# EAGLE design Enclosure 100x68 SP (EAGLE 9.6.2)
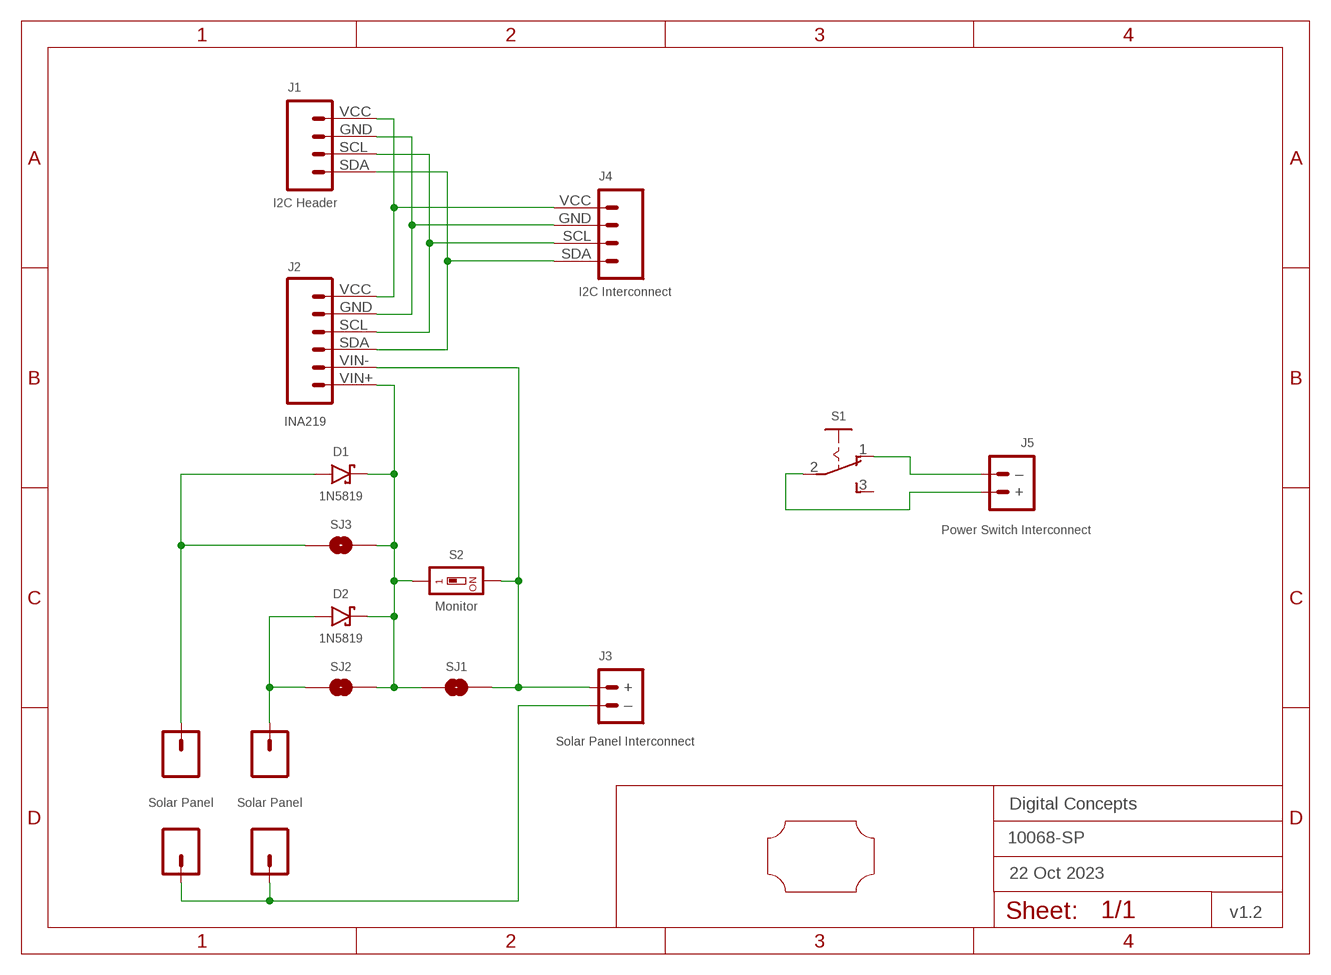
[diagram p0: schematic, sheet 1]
FRAME2 (FRAME_A5L-LOC): DATE: 22 Oct 2023; OWNER: Digital Concepts; TITLE: 10068-SP; VERSION: v1.2

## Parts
+  Solar Panel  PAD-SMD-GENERIC-SQUARE  [PAD-SMD-GENERIC]
+1  Solar Panel  PAD-SMD-GENERIC-SQUARE  [PAD-SMD-GENERIC]
-  Solar Panel  PAD-SMD-GENERIC-SQUARE  [PAD-SMD-GENERIC]
-1  Solar Panel  PAD-SMD-GENERIC-SQUARE  [PAD-SMD-GENERIC]
D1  1N5819  DIODE-SCHOTTKY-1N5819  [SOD-123]
D2  1N5819  DIODE-SCHOTTKY-1N5819  [SOD-123]
J1  I2C Header  HEADER-1X4-I2C  [CONN_04-I2C]
J2  INA219  INA219-I2C-MODULE  [CONN_06-INA219]
J3  Solar Panel Interconnect  JST-PH2.0-2-HORIZONTALJST-PTH-2  [JST-PH2.0-2-HORIZONTAL]
J4  I2C Interconnect  JST-PH2.0-4-I2C-HORIZONTAL  [JST-PH2.0-4-HORIZONTAL]
J5  Power Switch Interconnect  JST-PH2.0-2-HORIZONTALJST-PTH-2  [JST-PH2.0-2-HORIZONTAL]
S1  SWITCH-SLIDE-SPDT  [SWITCH-SPDT-PTH]
S2  Monitor  SWITCH-DIP-SWS001  [SMD-001]
SJ1  SJ  [SJ]
SJ2  SJ  [SJ]
SJ3  SJ  [SJ]
U$1  PROTO-34X22-SP  [PROTO-34X22-SP]

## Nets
GND: J1.GND J2.GND J4.GND
N$1: J1.SDA J2.SDA J4.SDA
N$2: J1.SCL J2.SCL J4.SCL
N$3: +1.P$1 D1.A SJ3.1
N$4: J2.VIN- J3.1(+) S2.2 SJ1.2
N$5: D1.C D2.C J2.VIN+ S2.1 SJ1.1 SJ2.2 SJ3.2
N$6: J5.1(+) S1.2(P)
N$7: -1.P$1 -.P$1 J3.2(–)
N$8: +.P$1 D2.A SJ2.1
N$9: J5.2(–) S1.1(O)
VCC: J1.VCC J2.VCC J4.VCC
Unconnected: S1.3(S)

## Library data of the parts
+ +1 - -1 = digitalconcepts:PAD-SMD-GENERIC-SQUARE: SMD Pad—Square
D1 D2 = digitalconcepts:DIODE-SCHOTTKY-1N5819: 1N5819 Schottky Diode SOD-123
J1 = digitalconcepts:HEADER-1X4-I2C: I2C Interface [Pin 1 Vcc] 4-Pin Header
J2 = digitalconcepts:INA219-I2C-MODULE: INA219 I2C Module
J3 J5 = digitalconcepts:JST-PH2.0-2-HORIZONTAL: PH2.0 2P Right Angle PCB Connector; PROD_ID: CONN-09863; SKU: PRT-09914
J4 = digitalconcepts:JST-PH2.0-4-I2C-HORIZONTAL: PH2.0 4P I2C Horizontal Connector
S1 = digitalconcepts:SWITCH-SLIDE-SPDT: Mini Sliding Switch SPDT
S2 = digitalconcepts:SWITCH-DIP-SWS001: SMD Dip Switch 1 pol.
SJ1-SJ3 = digitalconcepts:SJ: Solder Jumper
U$1 = digitalconcepts:PROTO-34X22-SP: 34 x 22 Prototyping board to fit an 100 x 68 enclosure—Solar panel support

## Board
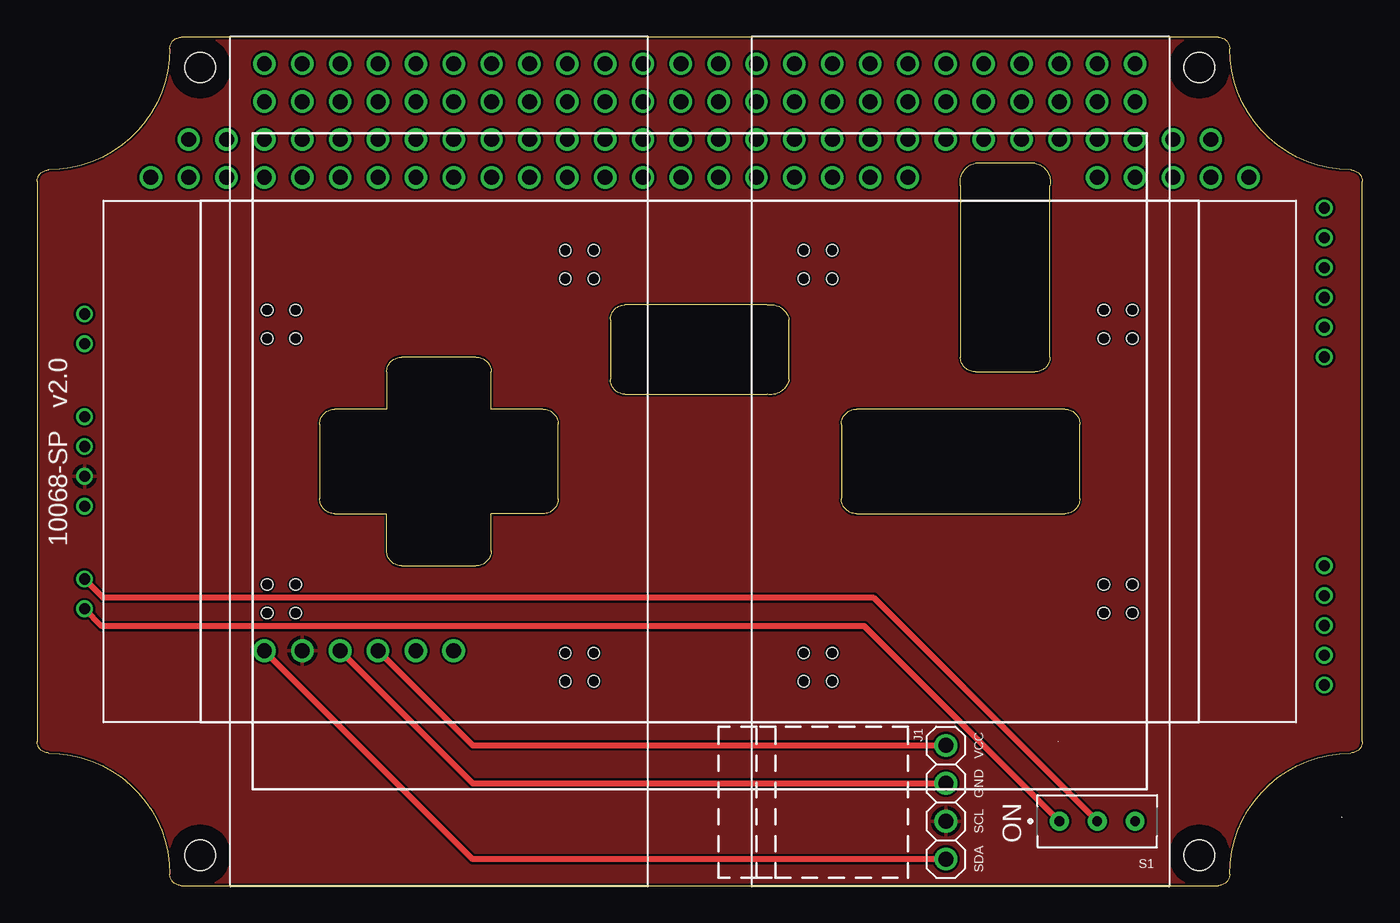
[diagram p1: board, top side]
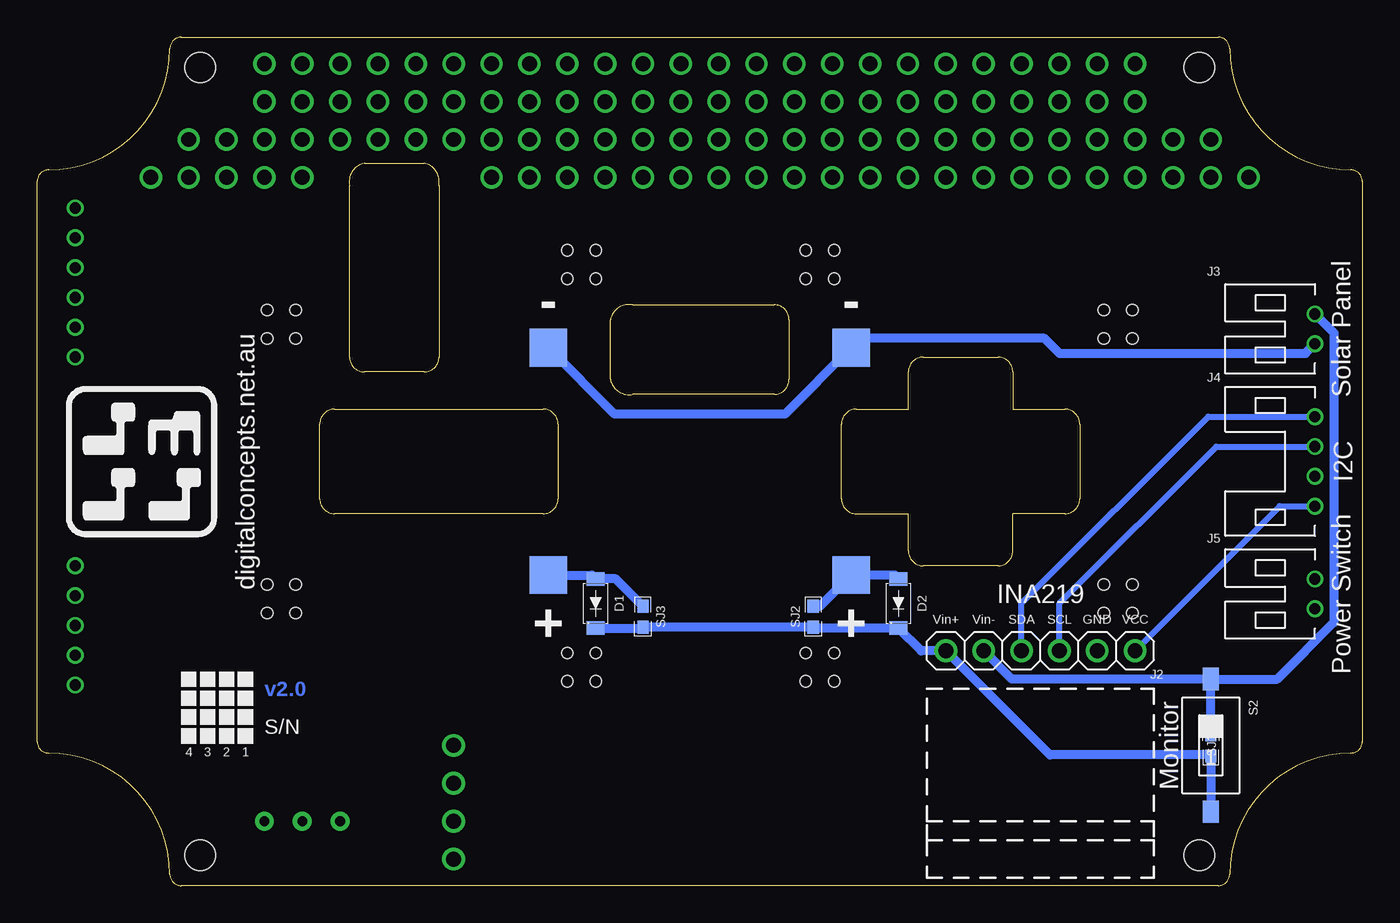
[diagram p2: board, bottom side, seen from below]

Size 88.9 x 56.9 mm. Coordinates in mm from the lower left corner, seen from the top.
Copper layers (1*16): Top 0.035mm / dielectric 1.5mm / Bottom 0.035mm
Design rules "default *": minimum track width 6mil, minimum drill 0.35mm, track to track 6mil, track to pad 6mil, pad to pad 6mil, via to via 6mil, smd to smd 6mil, copper to edge 6mil, drill to drill 6mil, minimum pad ring 1mil, minimum via ring 8mil, stop-mask expansion 4mil, vias tented up to drill 0mil, thermal gap 10mil

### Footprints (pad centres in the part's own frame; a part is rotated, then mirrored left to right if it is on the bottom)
PAD-SMD-GENERIC = smd 2.54 x 2.54: P$1 0,0
SOD-123 = smd 0.91 x 1.22: A -1.65,0; C 1.65,0
CONN_04-I2C = drill 1 pad 1.524: GND 2.54,0; SCL 5.08,0; SDA 7.62,0; VCC 0,0
CONN_06-INA219 = drill 1 pad 1.524: GND 2.54,0; SCL 5.08,0; SDA 7.62,0; VCC 0,0; VIN+ 12.7,0; VIN- 10.16,0
JST-PH2.0-2-HORIZONTAL = drill 0.75: 1 1,0; 2 -1,0
JST-PH2.0-4-HORIZONTAL = drill 0.75: GND -1,0; SCL 1,0; SDA 3,0; VCC -3,0
SWITCH-SPDT-PTH = drill 0.65 pad 1.27: 1 -2.54,0; 2 0,0; 3 2.54,0
SMD-001 = smd 1.1 x 1.5: 1 0,-4.45; 2 0,4.45
SJ = smd 0.864 x 0.762: 1 -0.711,0; 2 0.711,0
PROTO-34X22-SP = drill 0.75: P01-05 41.91,17; P01-06 41.91,15; P01-07 41.91,13; P01-08 41.91,11; P01-09 41.91,9; P01-10 41.91,7; P01-17 41.91,-7; P01-18 41.91,-9; P01-19 41.91,-11; P01-20 41.91,-13; P01-21 41.91,-15 | drill 1: P03-04 36.83,19.05; P04-03 34.29,21.59; P04-04 34.29,19.05; P05-03 31.75,21.59; P05-04 31.75,19.05; P06-01 29.21,26.67; P06-02 29.21,24.13; P06-03 29.21,21.59; P06-04 29.21,19.05; P07-01 26.67,26.67; P07-02 26.67,24.13; P07-03 26.67,21.59; P07-04 26.67,19.05; P08-01 24.13,26.67; P08-02 24.13,24.13; P08-03 24.13,21.59; P09-01 21.59,26.67; P09-02 21.59,24.13; P09-03 21.59,21.59; P10-01 19.05,26.67; P10-02 19.05,24.13; P10-03 19.05,21.59; P11-01 16.51,26.67; P11-02 16.51,24.13; P11-03 16.51,21.59; P12-01 13.97,26.67; P12-02 13.97,24.13; P12-03 13.97,21.59; P12-04 13.97,19.05; P13-01 11.43,26.67; P13-02 11.43,24.13; P13-03 11.43,21.59; P13-04 11.43,19.05; P14-01 8.89,26.67; P14-02 8.89,24.13; P14-03 8.89,21.59; P14-04 8.89,19.05; P15-01 6.35,26.67; P15-02 6.35,24.13; P15-03 6.35,21.59; P15-04 6.35,19.05; P16-01 3.81,26.67; P16-02 3.81,24.13; P16-03 3.81,21.59; P16-04 3.81,19.05; P17-01 1.27,26.67; P17-02 1.27,24.13; P17-03 1.27,21.59; P17-04 1.27,19.05; P18-01 -1.27,26.67; P18-02 -1.27,24.13; P18-03 -1.27,21.59; P18-04 -1.27,19.05; P19-01 -3.81,26.67; P19-02 -3.81,24.13; P19-03 -3.81,21.59; P19-04 -3.81,19.05; P20-01 -6.35,26.67; P20-02 -6.35,24.13; P20-03 -6.35,21.59; P20-04 -6.35,19.05; P21-01 -8.89,26.67; P21-02 -8.89,24.13; P21-03 -8.89,21.59; P21-04 -8.89,19.05; P22-01 -11.43,26.67; P22-02 -11.43,24.13; P22-03 -11.43,21.59; P22-04 -11.43,19.05; P23-01 -13.97,26.67; P23-02 -13.97,24.13; P23-03 -13.97,21.59; P23-04 -13.97,19.05; P24-01 -16.51,26.67; P24-02 -16.51,24.13; P24-03 -16.51,21.59; P24-04 -16.51,19.05; P25-01 -19.05,26.67; P25-02 -19.05,24.13; P25-03 -19.05,21.59; P25-04 -19.05,19.05; P26-01 -21.59,26.67; P26-02 -21.59,24.13; P26-03 -21.59,21.59; P26-04 -21.59,19.05; P27-01 -24.13,26.67; P27-02 -24.13,24.13; P27-03 -24.13,21.59; P27-04 -24.13,19.05; P28-01 -26.67,26.67; P28-02 -26.67,24.13; P28-03 -26.67,21.59; P28-04 -26.67,19.05; P29-01 -29.21,26.67; P29-02 -29.21,24.13; P29-03 -29.21,21.59; P29-04 -29.21,19.05; P30-03 -31.75,21.59; P30-04 -31.75,19.05; P31-03 -34.29,21.59; P31-04 -34.29,19.05; P32-04 -36.83,19.05 | hole 2.032: 33.528,-26.416; -33.528,-26.416; -33.528,26.416; 33.528,26.416 | hole 0.75: 29.02,-10.16; 27.115,-10.16; 27.115,-8.255; 29.02,-8.255; 29.02,8.255; 27.115,8.255; 27.115,10.16; 29.02,10.16; -27.115,8.255; -29.02,8.255; -29.02,10.16; -27.115,10.16; -27.115,-10.16; -29.02,-10.16; -29.02,-8.255; -27.115,-8.255; -7.115,12.255; -9.02,12.255; -9.02,14.16; -7.115,14.16; 8.885,12.255; 6.98,12.255; 6.98,14.16; 8.885,14.16; 8.885,-14.745; 6.98,-14.745; 6.98,-12.84; 8.885,-12.84; -7.115,-14.745; -9.02,-14.745; -9.02,-12.84; -7.115,-12.84

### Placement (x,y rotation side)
+  34.29,20.83 180 bottom
+1  54.61,20.83 180 bottom
-  34.29,36.07 180 bottom
-1  54.61,36.07 180 bottom
D1  51.44,18.92 270 bottom
D2  31.12,18.92 270 bottom
J1  60.96,1.78 90 top
J2  15.24,15.75 180 bottom
J3  3.18,37.34 90 bottom
J4  3.18,28.45 90 bottom
J5  3.18,19.56 90 bottom
S1  71.12,4.32 0 top
S2  10.16,9.4 0 bottom
SJ1  10.16,9.4 90 bottom
SJ2  36.83,18.03 270 bottom
SJ3  48.26,18.03 270 bottom
U$1  44.45,28.45 0 top

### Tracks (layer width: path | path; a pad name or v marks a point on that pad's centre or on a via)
$X0
  cutout Bottom: 77.98,0 arc180 77.98,4.06 arc180
$X1
  cutout Bottom: 10.92,0 arc180 10.92,4.06 arc180
$X2
  cutout Bottom: 10.92,52.83 arc180 10.92,56.9 arc180
$X3
  cutout Bottom: 77.98,52.83 arc180 77.98,56.9 arc180
$X4
  cutout Top: 77.98,0 arc180 77.98,4.06 arc180
$X5
  cutout Top: 10.92,0 arc180 10.92,4.06 arc180
$X6
  cutout Top: 10.92,52.83 arc180 10.92,56.9 arc180
$X7
  cutout Top: 77.98,52.83 arc180 77.98,56.9 arc180
GND
  pour Top: 90.17,-1.4 -1.27,-1.4 -1.27,58.29 90.17,58.29
N$1
  Top 0.406: J2.SDA 29.21,9.4 J1.SDA
  Bottom 0.406: J2.SDA 22.86,18.92 10.34,31.45 J4.SDA
N$2
  Top 0.406: J1.SCL 29.21,6.86 J2.SCL
  Bottom 0.406: J2.SCL 20.32,18.92 9.8,29.45 J4.SCL
N$3
  Bottom 0.61: +1.P$1 51.69,20.83 D1.A 50.09,20.57 SJ3.1
N$4
  Bottom 0.61: J3.1 1.91,37.07 1.91,17.66 5.72,13.85 S2.2 | SJ1.2 S2.2 | S2.2 23.5,13.85 J2.VIN-
N$5
  Bottom 0.61: S2.1 SJ1.1 10.24,8.76 20.96,8.76 J2.VIN+ 29.59,15.75 D2.C 36.78,17.27 SJ2.2 SJ3.2 48.31,17.27 D1.C
N$6
  Top 0.406: S1.2 56.13,19.3 4.43,19.3 J5.1
N$7
  Bottom 0.61: J3.2 3.81,35.7 20.32,35.7 21.32,36.7 33.66,36.7 -.P$1 38.73,31.62 50.16,31.62 -1.P$1
N$8
  Bottom 0.61: D2.A 31.37,20.83 +.P$1 36.37,18.75 SJ2.1
N$9
  Top 0.406: S1.1 55.5,17.4 4.33,17.4 J5.2
VCC
  Top 0.406: J1.VCC 29.21,1.78 J2.VCC
  Bottom 0.406: J2.VCC 5.54,25.45 J4.VCC

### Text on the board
Bottom: v2.0
tPlace: 10068-SP v2.0 | VCC | GND | SCL | ON | SDA
bPlace: digitalconcepts.net.au | VCC | GND | SCL | SDA | Vin- | Vin+ | S/N | 1 | 2 | 3 | 4
bNames: - | Solar Panel | I2C | Power Switch | +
